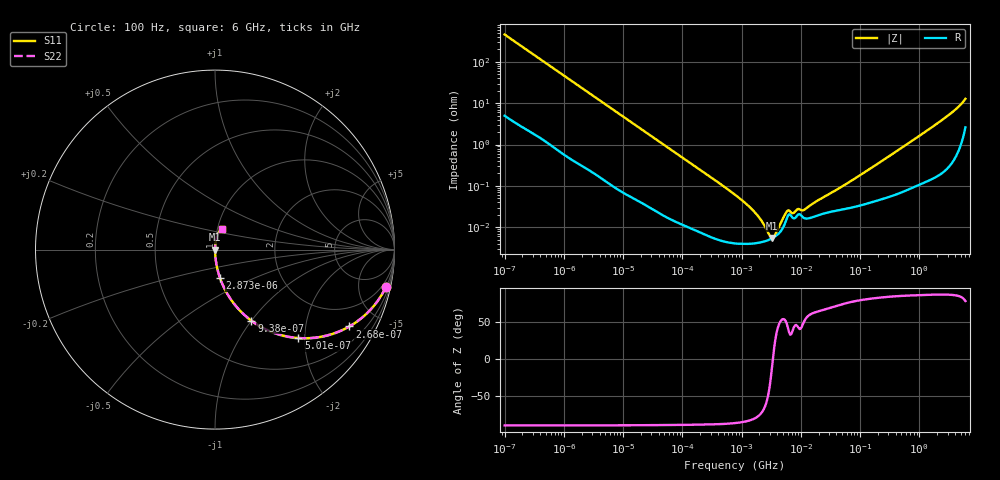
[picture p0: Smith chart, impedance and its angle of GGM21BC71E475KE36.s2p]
!Murata Part Number: GGM21BC71E475KE36
!These Parameters are Measured in Series Mode Connection
!Data Generated on Jun 19, 2026
!  o--ll--o
!Port1  Port2
!  o------o
!Operation Temp=25[degC], DC Bias Voltage=0[V]
!Freq. Start=100[Hz] Stop=6[GHz] 401[Steps]
# Hz S RI R 50
!Freq.(Hz) S11(Real) S11(Imag) S21(Real) S21(Imag) S12(Real) S12(Imag) S22(Real) S22(Imag)
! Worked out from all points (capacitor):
!   401 points, 100 Hz to 6 GHz, reference 50 ohm
!   read as one part in series: C = 3.44 uF near 109 Hz
!   lowest |Z| = 5.49 mohm at 3.246 MHz (marker M1)
!   series resonance near 3.376 MHz, so ESL is about 650 pH
!   S11 on the Smith chart (normalised r, x): 100 Hz: 1.10, -9.22; 268 Hz: 1.04, -3.47; 501 Hz: 1.02, -1.86; 938 Hz: 1.01, -1.00; 2.873 kHz: 1.00, -0.33; 6 GHz: 1.05, +0.25
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100  0.953 -0.2062  0.047 0.2062  0.047 0.2062  0.953 -0.2062
164  0.8861 -0.3122  0.1139 0.3122  0.1139 0.3122  0.8861 -0.3122
268  0.7477 -0.4284  0.2523 0.4284  0.2523 0.4284  0.7477 -0.4284
501  0.4648 -0.4926  0.5352 0.4926  0.5352 0.4926  0.4648 -0.4926
938  0.2029 -0.3961  0.7971 0.3961  0.7971 0.3961  0.2029 -0.3961
2008  0.0548 -0.2212  0.9452 0.2212  0.9452 0.2212  0.0548 -0.2212
2873  0.0284 -0.1596  0.9716 0.1596  0.9716 0.1596  0.0284 -0.1596
8416  0.004 -0.0565  0.996 0.0565  0.996 0.0565  0.004 -0.0565
40335  0.000365 -0.012  0.9996 0.012  0.9996 0.012  0.000365 -0.012
774597  4.1e-05 -0.000611  1 0.000611  1 0.000611  4.1e-05 -0.000611
1516199  4.03e-05 -0.000264  1 0.000264  1 0.000264  4.03e-05 -0.000264
2481164  4.59e-05 -9.42e-05  1 9.42e-05  1 9.42e-05  4.59e-05 -9.42e-05
3245845  5.36e-05 -1.2e-05  0.9999 1.2e-05  0.9999 1.2e-05  5.36e-05 -1.2e-05
4246196  7.08e-05 7.38e-05  0.9999 -7.38e-05  0.9999 -7.38e-05  7.08e-05 7.38e-05
6075234  0.000191 0.000171  0.9998 -0.000171  0.9998 -0.000171  0.000191 0.000171
7266822  0.00017 0.000134  0.9998 -0.000134  0.9998 -0.000134  0.00017 0.000134
9090158  0.000205 0.000188  0.9998 -0.000188  0.9998 -0.000188  0.000205 0.000188
1.137099e7  0.000167 0.000204  0.9998 -0.000204  0.9998 -0.000204  0.000167 0.000204
1.555665e7  0.000174 0.000321  0.9998 -0.000321  0.9998 -0.000321  0.000174 0.000321
3.124326e8  0.000572 0.00525  0.9994 -0.00525  0.9994 -0.00525  0.000572 0.00525
2.562649e9  0.00389 0.0415  0.9961 -0.0415  0.9961 -0.0415  0.00389 0.0415
6e9  0.0396 0.117  0.9604 -0.117  0.9604 -0.117  0.0396 0.117
